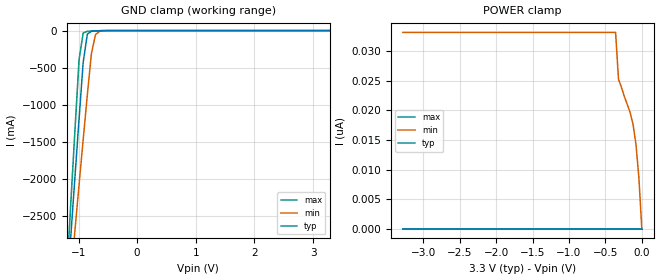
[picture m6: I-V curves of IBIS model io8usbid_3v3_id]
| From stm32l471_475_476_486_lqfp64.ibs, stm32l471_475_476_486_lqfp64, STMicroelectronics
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|   Model io8usbid_3v3_id
[Model]  io8usbid_3v3_id
Model_type Input
Polarity   Non-Inverting
Vinl =   0.540000V
Vinh =   1.260000V
C_comp   2.116400pF   2.092900pF   2.152900pF
[Temperature Range]   25.000000   0.125000k   -40.000000
[Pullup Reference]   3.300000V   2.700000V   3.600000V
[Pulldown Reference]   0.0V   0.0V   0.0V
[POWER Clamp Reference]   3.300000V   2.700000V   3.600000V
[GND Clamp Reference]   0.0V   0.0V   0.0V
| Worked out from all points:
|   GND clamp passes 1 mA (typ) near -0.59 V on its own axis
[GND_clamp]
|Voltage   I(typ)   I(min)   I(max)
-3.3V     -9.914A    -9.595A    -9.188A
-1.2V     -3.541A    -3.911A    -3.279A
-1.13V    -2.75A     -3.295A    -2.301A
-1.06V    -1.963A    -2.68A     -1.33A
-990mV    -1.183A    -2.069A    -386.7mA
-920mV    -424.7mA   -1.463A    -31.42mA
-850mV    -49.12mA   -868.7mA   -10.48mA
-780mV    -9.121mA   -308.3mA   -6.715mA
-710mV    -3.648mA   -53.81mA   -3.986mA
-640mV    -1.726mA   -11.03mA   -1.885mA
-430mV    -22.46uA   -116.8uA   -9.748uA
3.28V     0A         0A         0A
[POWER_clamp]
|Voltage   I(typ)   I(min)   I(max)
-3.28V    0A         33.18nA    0A
-360mV    0A         33.18nA    0A
-320mV    0A         25.29nA    0A
-280mV    0A         23.92nA    0A
-240mV    0A         22.34nA    0A
-200mV    0A         21.02nA    0A
-160mV    0A         19.6nA     0A
-120mV    0A         17.61nA    0A
-80mV     0A         14.24nA    0A
-40mV     0A         8.614nA    0A
0V        0A         0A         0A
